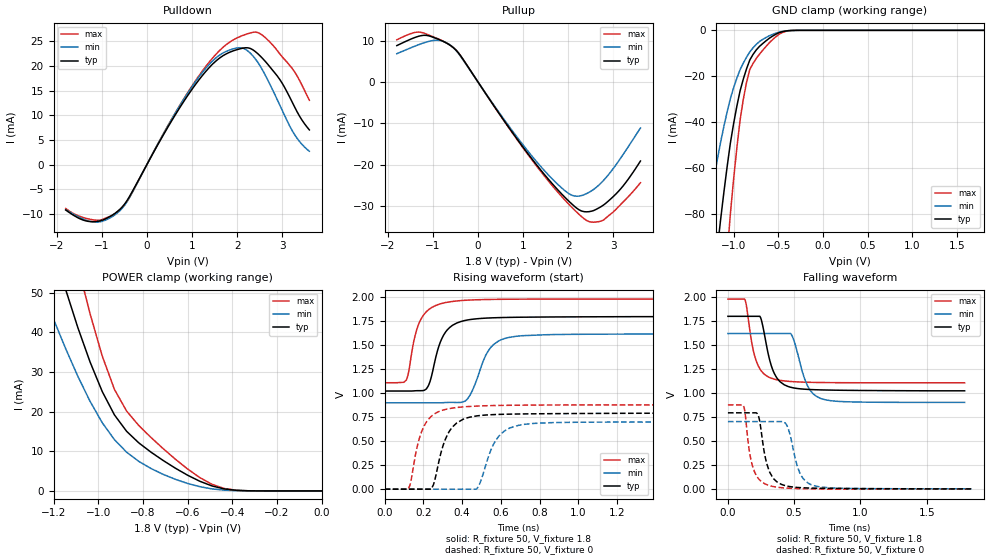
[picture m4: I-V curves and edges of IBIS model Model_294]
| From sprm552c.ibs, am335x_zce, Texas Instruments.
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| Model based on original model for BCSHTLTCSCDVPBFZ_SSDHV
|   Sub model SR00_6MA_10PER_1P8
[model]   Model_294
|[Description]  [1.8V-3-STATE-NOTERM-SR00:6MA, IND, 10%]
|   Fastest slew rate (SR[1:0] = "00"), 1.33 * RExt = 0.750 * Iout
|   (I[2:0] = "001"), 6mA nominal with Rext = 50R,ODT off (ODT[1:0]
|   = "00") CMOS mode,Industrial temperature range (-40C to 125C,
|   25C nominal),10% power supply tolerance
|[Input Load]   NOTERM
|[Output Drive] SR00:6MA
|Voltage   1.8V
|Mode   3-STATE
Model_type   3-state
Polarity   Non-Inverting
Enable   Active-Low
Cref =  15pF
Rref =  100.0000M
Vref =  0V
Vmeas =  0.9
C_comp   1.851324p   1.663768p   1.973575p
[Temperature Range]   25   125   -40
[Voltage Range]   1.8   1.62   1.98
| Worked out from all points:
|   slope of the pulldown table from 0 to 0.27 V, typ, clamps not added: 60.1 ohm
|   slope of the pullup table from 0 to 0.27 V, typ, clamps not added: 60.8 ohm
|   GND clamp passes 1 mA (typ) near -0.49 V on its own axis
|   POWER clamp passes 1 mA (typ) near -0.47 V on its own axis
|   rising waveform, R_fixture 50, V_fixture 1.8: 20-80 % time 74.6ps typ, 90.4ps min, 68.7ps max; typ from 1.02 V to 1.8 V
|   rising waveform, R_fixture 50, V_fixture 0: 20-80 % time 78.2ps typ, 87.9ps min, 73.1ps max; typ from 0 V to 0.791 V
|   falling waveform, R_fixture 50, V_fixture 1.8: 20-80 % time 89.4ps typ, 99.6ps min, 79.2ps max; typ from 1.8 V to 1.02 V
|   falling waveform, R_fixture 50, V_fixture 0: 20-80 % time 73.5ps typ, 83ps min, 66ps max; typ from 0.795 V to 0.003 V
[POWER_clamp]
-1.8V     194.9mA    137.1mA    262.8mA
-1.236V   68.49mA    48.51mA    92.67mA
-1.145V   50.76mA    35.86mA    69.65mA
-1.127V   47.56mA    33.54mA    65.34mA
-1.055V   35.4mA     24.69mA    48.69mA
-981.8mV  25.06mA    17.2mA     34.01mA
-927.3mV  19.17mA    12.93mA    25.61mA
-872.7mV  15.03mA    9.767mA    20.12mA
-818.2mV  12.12mA    7.45mA     16.5mA
-654.5mV  5.738mA    2.93mA     8.003mA
-436.4mV  508.2uA    199.4uA    613uA
0V        2.273nA    15.95nA    16.67nA
[Pulldown]
-1.8V     -9.241mA   -9.161mA   -8.932mA
-1.145V   -11.6mA    -11.72mA   -11.3mA
-545.5mV  -8.602mA   -8.855mA   -8.702mA
545.5mV   8.836mA    9.123mA    9.182mA
1.091V    16.44mA    17.01mA    17.21mA
1.527V    21.01mA    21.64mA    22.36mA
1.964V    23.24mA    23.61mA    25.56mA
2.291V    23.58mA    22.62mA    26.72mA
2.618V    21mA       18.23mA    25.82mA
2.945V    17.26mA    12.06mA    22.47mA
3.218V    12.7mA     6.898mA    19.53mA
3.6V      7.029mA    2.696mA    13.05mA
[Pullup]
-1.8V     8.832mA    6.868mA    10.25mA
-1.2V     11.33mA    9.506mA    11.86mA
-872.7mV  10.35mA    10.11mA    10.42mA
-600mV    8.779mA    8.832mA    8.794mA
-381.8mV  6.289mA    6.153mA    6.32mA
1.2V      -18.71mA   -18.02mA   -18.96mA
1.745V    -25.88mA   -24.59mA   -26.41mA
2.127V    -30.05mA   -27.62mA   -30.92mA
2.455V    -31.44mA   -26.78mA   -33.81mA
2.727V    -30.21mA   -24.47mA   -33.71mA
3.164V    -25.87mA   -18.41mA   -29.67mA
3.6V      -19.15mA   -11.15mA   -24.41mA
[GND_clamp]
-1.8V     -346.1mA   -209.3mA   -568.3mA
-1.327V   -149.7mA   -89.03mA   -250.9mA
-1.291V   -135.6mA   -80.47mA   -227.5mA
-1.145V   -82.35mA   -48.67mA   -137.7mA
-1.073V   -59.44mA   -35.55mA   -97.96mA
-1.036V   -49.1mA    -29.72mA   -79.9mA
-927.3mV  -26.31mA   -17.11mA   -38.99mA
-854.5mV  -16.67mA   -11.64mA   -22.56mA
-818.2mV  -12.86mA   -9.351mA   -16.98mA
-672.7mV  -5.705mA   -3.913mA   -8.624mA
-381.8mV  -120.4uA   -129uA     -167.4uA
1.8V      2.273nA    454nA      6.646nA
[Ramp]
dV/dt_f 0.47395249/90.031512p  0.4413209/0.10093358n 0.52829257/79.326199p
dV/dt_r 0.48238973/79.317359p 0.43064166/88.69452p   0.5307826/72.940678p
R_load = 50
[Rising Waveform]
R_fixture = 50
V_fixture = 1.8
V_fixture_min = 1.62
V_fixture_max = 1.98
0s        1.022V     899.3mV    1.108V
112.9ps   1.022V     899.3mV    1.139V
165.4ps   1.025V     899.3mV    1.659V
215.3ps   1.044V     899.3mV    1.848V
306ps     1.61V      901.3mV    1.94V
421.4ps   1.76V      926.6mV    1.968V
453.3ps   1.77V      1.029V     1.971V
534.3ps   1.783V     1.438V     1.976V
637.6ps   1.789V     1.579V     1.978V
1.787ns   1.797V     1.616V     1.98V
[Rising Waveform]
R_fixture = 50
V_fixture = 0
V_fixture_min = 0
V_fixture_max = 0
0s        0V         0V         0V
121.9ps   0V         0V         0V
184.9ps   0V         0V         565.6mV
240.4ps   0V         0V         757.7mV
312.1ps   512.4mV    0V         829.7mV
371.7ps   688.8mV    0V         850.4mV
474.3ps   762.7mV    0V         865.2mV
572.7ps   777.4mV    504.4mV    871.3mV
691.9ps   783mV      665.1mV    874.7mV
1.839ns   791.5mV    699.7mV    877.7mV
[Falling Waveform]
R_fixture = 50
V_fixture = 1.8
V_fixture_min = 1.62
V_fixture_max = 1.98
0s        1.8V       1.621V     1.98V
130.3ps   1.8V       1.621V     1.967V
190.1ps   1.8V       1.621V     1.455V
241.3ps   1.8V       1.621V     1.253V
326.9ps   1.288V     1.621V     1.156V
389.4ps   1.125V     1.621V     1.134V
474.2ps   1.061V     1.621V     1.121V
602.2ps   1.039V     1.073V     1.113V
701.9ps   1.034V     943.9mV    1.111V
1.787ns   1.024V     903.5mV    1.107V
[Falling Waveform]
R_fixture = 50
V_fixture = 0
V_fixture_min = 0
V_fixture_max = 0
0s        795mV      703.8mV    877.2mV
121.9ps   795mV      703.8mV    852.6mV
170.8ps   795mV      703.8mV    327mV
221.3ps   787.1mV    703.8mV    127.4mV
279.5ps   347.5mV    703.8mV    55.58mV
311.1ps   190.5mV    703.8mV    37.93mV
441.6ps   33.79mV    672.2mV    11.34mV
540.5ps   16.46mV    176.3mV    5.814mV
650.7ps   10.71mV    36.43mV    3.05mV
1.839ns   2.842mV    3.966mV    0V
